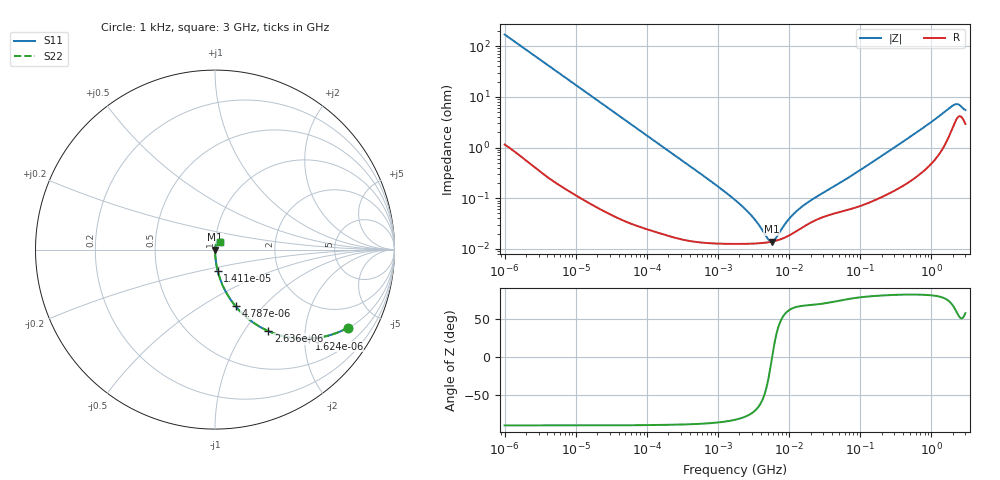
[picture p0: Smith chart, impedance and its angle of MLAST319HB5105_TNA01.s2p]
! MLAST319HB5105_TNA01  S-PARAMETER MODEL  ( Standard Model )
! Model Generated by TAIYO YUDEN Corporation (http://www.ty-top.com)
! Version 1.0
! TAIYO YUDEN Control No. 220601
! Copyright(c) 2009 TAIYO YUDEN CO.,LTD. All Rights Reserved.
! Product Description (link to TY-COMPAS)
! https://ds.yuden.co.jp/TYCOMPAS/or/detail?pn=MLAST319HB5105KTNA01&u=M
! Products Name : Multilayer Ceramic Capacitors
! Characteristics :
!  Capacitance : 1 [uF] , Rated Voltage : 25 [V] , TCC : B / X5R
!  Case Size : 3.2 x 1.6 / 0.126 x 0.063 [mm/inch] , Thickness : 0.85 / 0.033 [mm/inch]
!  (Conditions: Temperature = 25 [degC] , DC Bias Voltage = 0 [V])
! External Node Assignments :
!  1  o---| |---o  2
! GND o---------o GND
! Frequency Range : 1kHz  -  3GHz  [ 401 STEP ]
# MHZ S RI R 50
! Freq[MHz].  S11 Real  S11 Imag  S21 Real  S21 Imag  S12 Real  S12 Imag  S22 Real  S22 Imag
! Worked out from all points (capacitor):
!   401 points, 1 kHz to 3 GHz, reference 50 ohm
!   read as one part in series: C = 936 nF near 1.077 kHz
!   lowest |Z| = 13.9 mohm at 5.711 MHz (marker M1)
!   series resonance near 5.753 MHz, so ESL is about 820 pH
!   S11 on the Smith chart (normalised r, x): 1 kHz: 1.02, -3.40; 1.624 kHz: 1.01, -2.10; 2.636 kHz: 1.01, -1.29; 4.787 kHz: 1.00, -0.71; 14.12 kHz: 1.00, -0.24; 3 GHz: 1.06, +0.09
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0.001  0.7411 -0.4347  0.2589 0.4347  0.2589 0.4347  0.7411 -0.4347
0.001624  0.5236 -0.4961  0.4764 0.4961  0.4764 0.4961  0.5236 -0.4961
0.002636  0.2964 -0.4535  0.7036 0.4535  0.7036 0.4535  0.2964 -0.4535
0.004787  0.1146 -0.3155  0.8854 0.3155  0.8854 0.3155  0.1146 -0.3155
0.01216  0.0204 -0.1381  0.9796 0.1381  0.9796 0.1381  0.0204 -0.1381
0.014115  0.0154 -0.1196  0.9846 0.1196  0.9846 0.1196  0.0154 -0.1196
0.037214  0.00255 -0.0462  0.9974 0.0462  0.9974 0.0462  0.00255 -0.0462
0.147855  0.000343 -0.0117  0.9997 0.0117  0.9997 0.0117  0.000343 -0.0117
1.732051  0.000126 -0.000917  0.9999 0.000917  0.9999 0.000917  0.000126 -0.000917
2.919173  0.000127 -0.000445  0.9999 0.000445  0.9999 0.000445  0.000127 -0.000445
3.651041  0.000129 -0.000286  0.9999 0.000286  0.9999 0.000286  0.000129 -0.000286
4.919932  0.000134 -9.56e-05  0.9999 9.56e-05  0.9999 9.56e-05  0.000134 -9.56e-05
5.711239  0.000139 -4.33e-06  0.9999 4.33e-06  0.9999 4.33e-06  0.000139 -4.33e-06
6.387174  0.000144 6.38e-05  0.9999 -6.38e-05  0.9999 -6.38e-05  0.000144 6.38e-05
8.933959  0.000171 0.000273  0.9998 -0.000273  0.9998 -0.000273  0.000171 0.000273
11.1738  0.000202 0.00042  0.9998 -0.00042  0.9998 -0.00042  0.000202 0.00042
21.06097  0.000342 0.000881  0.9997 -0.000881  0.9997 -0.000881  0.000342 0.000881
64.45588  0.000587 0.00236  0.9994 -0.00236  0.9994 -0.00236  0.000587 0.00236
256.0921  0.00132 0.0085  0.9987 -0.0085  0.9987 -0.0085  0.00132 0.0085
1990.675  0.0279 0.0591  0.9721 -0.0591  0.9721 -0.0591  0.0279 0.0591
2310.849  0.0403 0.0561  0.9597 -0.0561  0.9597 -0.0561  0.0403 0.0561
3000  0.0303 0.044  0.9697 -0.044  0.9697 -0.044  0.0303 0.044
